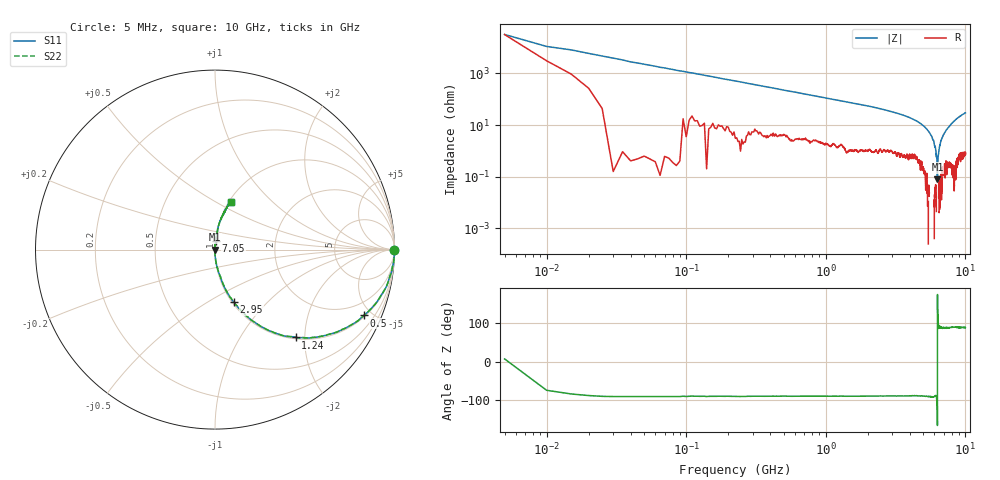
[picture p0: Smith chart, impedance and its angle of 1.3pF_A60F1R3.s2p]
! Amotech Co.,Ltd.
! http://www.amotech.co.kr/
! Part Number: A60F1R3
! These Parameters are Measured in Series Mode Connection
! Operation Temp=25[degC], DC Bias Voltage=0[V]
! Freq. Start=5[MHz] Stop=10[GHz], 2000[Steps]
! Date: Monday, July 20, 2020, 03:13:17
# GHZ S RI R 50.000000
!Freq.(Hz) S11(Real) S11(Imag) S21(Real) S21(Imag) S12(Real) S12(Imag) S22(Real) S22(Imag)
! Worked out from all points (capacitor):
!   2000 points, 5 MHz to 10 GHz, reference 50 ohm
!   read as one part in series: C = 1.41 pF near 55 MHz
!   lowest |Z| = 81 mohm at 6.305 GHz (marker M1)
!   series resonance near 6.308 GHz, so ESL is about 450 pH
!   S11 on the Smith chart (normalised r, x): 5 MHz: open; 500 MHz: 1.09, -4.48; 1.24 GHz: 1.03, -1.80; 2.95 GHz: 1.02, -0.66; 7.05 GHz: 1.01, +0.09; 10 GHz: 1.02, +0.59
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0.005  0.9969 0.00039  0.0031 -0.00039  0.0031 -0.00039  0.9969 0.00039
0.07  0.9962 -0.0613  0.00379 0.0613  0.00379 0.0613  0.9962 -0.0613
0.135  0.9847 -0.116  0.0153 0.116  0.0153 0.116  0.9847 -0.116
0.28  0.9394 -0.2318  0.0606 0.2318  0.0606 0.2318  0.9394 -0.2318
0.5  0.8293 -0.3666  0.1707 0.3666  0.1707 0.3666  0.8293 -0.3666
1.24  0.4494 -0.4891  0.5506 0.4891  0.5506 0.4891  0.4494 -0.4891
1.675  0.309 -0.4548  0.691 0.4548  0.691 0.4548  0.309 -0.4548
2.95  0.1065 -0.2937  0.8935 0.2937  0.8935 0.2937  0.1065 -0.2937
3.34  0.0753 -0.2489  0.9247 0.2489  0.9247 0.2489  0.0753 -0.2489
5.005  0.0106 -0.0919  0.9894 0.0919  0.9894 0.0919  0.0106 -0.0919
5.545  0.00221 -0.0498  0.9978 0.0498  0.9978 0.0498  0.00221 -0.0498
5.92  0.000308 -0.0252  0.9997 0.0252  0.9997 0.0252  0.000308 -0.0252
6.13  0.000549 -0.0107  0.9995 0.0107  0.9995 0.0107  0.000549 -0.0107
6.215  -0.000264 -0.00613  1 0.00613  1 0.00613  -0.000264 -0.00613
6.27  -0.000962 -0.00269  1.001 0.00269  1.001 0.00269  -0.000962 -0.00269
6.305  -0.000782 -0.000214  1.001 0.000214  1.001 0.000214  -0.000782 -0.000214
6.33  -0.00142 0.00203  1.001 -0.00203  1.001 -0.00203  -0.00142 0.00203
6.435  0.000643 0.00827  0.9994 -0.00827  0.9994 -0.00827  0.000643 0.00827
6.67  0.00162 0.0238  0.9984 -0.0238  0.9984 -0.0238  0.00162 0.0238
7.05  0.00492 0.0462  0.9951 -0.0462  0.9951 -0.0462  0.00492 0.0462
8.335  0.0219 0.1442  0.9781 -0.1442  0.9781 -0.1442  0.0219 0.1442
10  0.0871 0.2679  0.9129 -0.2679  0.9129 -0.2679  0.0871 0.2679
